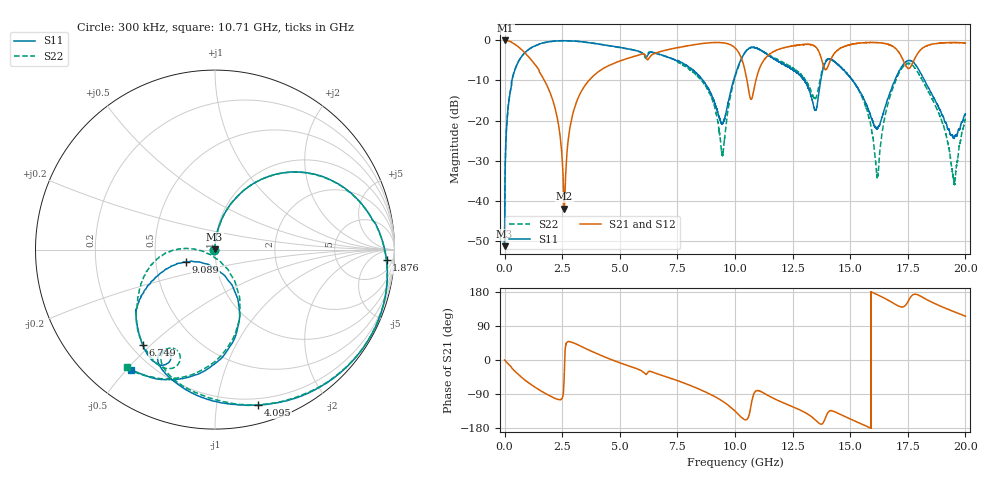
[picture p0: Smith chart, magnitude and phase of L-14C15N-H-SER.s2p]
!{L-14C15N}
!Johanson Technology Inc.
!www.johansontechnology.com
!Test Board Conditions:
!Substrate Type  RO4350B
!Substrate Thickness  20 mil
!Substrate Dk  3.66
!TL Type: GCPW
!TL Trace Width  36 mil
!TL Gap  12 mil
!Electrode orientation  Horizontal
!DUT TOPOLOGY	SERIES
!Mounting Pad LxW  26x36 mil
! Created Sun Jun 20 13:01:39 2021
# hz S ma R 50
! 2 Port Network Data from SP1.SP block
! freq  magS11  angS11  magS21  angS21  magS12  angS12  magS22  angS22
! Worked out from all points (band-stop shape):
!   20001 points, 300 kHz to 20 GHz, reference 50 ohm
!   highest |S21| = -0.01 dB at 33.3 MHz (marker M1); lowest = -42.0 dB at 2.595 GHz (marker M2)
!   |S21| within 3 dB of the highest: 6.63 GHz to 10.16 GHz (3.528 GHz wide, 42 % of centre); 14.35 GHz to 17.12 GHz (2.771 GHz wide, 17.6 % of centre)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
!   lowest |S11| = -51.4 dB at 1.3 MHz (marker M3), VSWR 1.01, Z = 49.8 + j0.144 ohm
!   |S11| at or under -10 dB: 8.614 GHz to 9.938 GHz (1.324 GHz wide, 14.3 % of centre); 15.12 GHz to 16.93 GHz (1.816 GHz wide, 11.3 % of centre); 18.23 GHz to end of sweep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
!   |S22| runs from -51.0 to -0.1 dB; largest |S21 - S12| = 0.013
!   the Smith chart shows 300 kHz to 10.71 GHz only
!   S11 on the Smith chart (normalised r, x): 300 kHz: 0.99, -0.00; 1.876 GHz: 15, -22; 4.095 GHz: 0.14, -1.31; 6.749 GHz: 0.25, -0.47; 9.089 GHz: 0.71, -0.10; 10.71 GHz: 0.13, -0.51
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300000  0.003826 -162.0  0.997 0.1  0.9956 0.2  0.003879 -156.0
1300000  0.002704 147.8  0.9977 -0.0  0.9977 -0.0  0.002835 145.0
3.33e7  0.0336 88.3  0.9992 -2.3  0.999 -2.3  0.03376 88.2
4.203e8  0.4091 61.0  0.9045 -27.9  0.904 -27.9  0.4106 60.9
1.8763e9  0.9575 -3.6  0.2595 -91.9  0.26 -91.8  0.957 -3.8
2.5953e9  0.9921 -28.0  0.007937 -20.4  0.008012 -20.6  0.9921 -28.0
3.3343e9  0.9639 -52.4  0.2319 35.6  0.233 35.6  0.9624 -51.8
4.0953e9  0.8993 -74.5  0.4115 14.5  0.4108 14.4  0.9008 -73.4
6.6673e9  0.6786 -125.5  0.7129 -37.4  0.7142 -37.2  0.6742 -125.2
6.7493e9  0.6669 -127.1  0.724 -39.0  0.7253 -38.8  0.664 -127.0
9.0893e9  0.1766 -157.2  0.94 -95.6  0.941 -95.7  0.158 177.6
9.4683e9  0.09274 -107.3  0.9341 -109.0  0.9349 -109.2  0.0375 -115.2
1.00003e10  0.3635 -68.2  0.8076 -134.6  0.8068 -134.6  0.3473 -66.5
1.07093e10  0.8168 -125.4  0.184 -115.4  0.1861 -115.7  0.8185 -127.3
1.17773e10  0.5657 175.1  0.7494 -104.3  0.7498 -104.4  0.589 169.8
1.33343e10  0.1871 143.1  0.8823 -150.2  0.8801 -150.3  0.218 148.0
1.48993e10  0.374 124.2  0.8719 -153.1  0.8677 -152.9  0.3727 123.6
1.61723e10  0.07891 166.0  0.9399 172.4  0.9398 172.5  0.01967 166.4
1.66673e10  0.198 -149.3  0.8914 157.2  0.8859 157.3  0.1755 -131.3
1.77733e10  0.5257 133.0  0.571 173.5  0.5766 174.0  0.465 123.5
1.95003e10  0.05965 138.1  0.9402 127.7  0.9447 127.7  0.01722 108.2
2e10  0.1205 -175.6  0.9286 115.6  0.923 115.4  0.1034 -179.0
